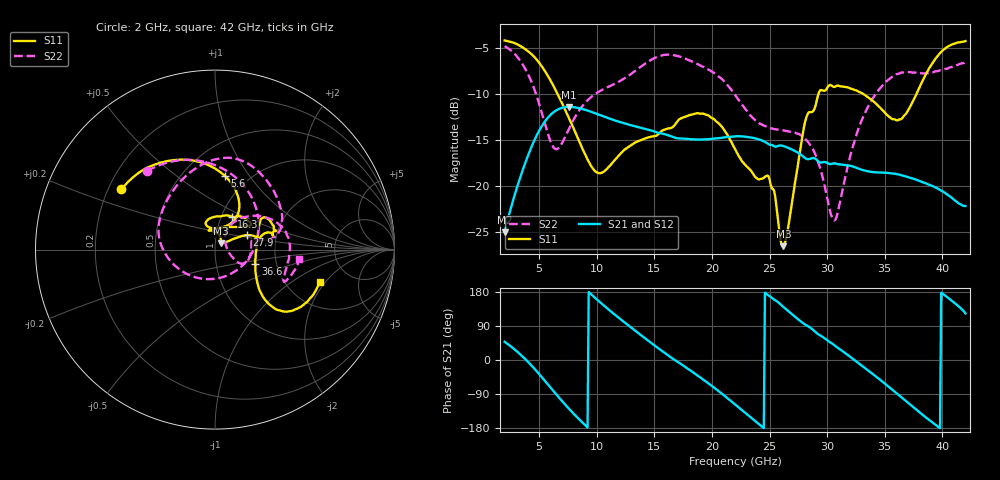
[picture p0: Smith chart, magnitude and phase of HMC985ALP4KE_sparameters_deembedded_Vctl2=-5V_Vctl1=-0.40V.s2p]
!s2p File: Measurements: S11, S21, S12, S22
# GHz S dB R 50.0
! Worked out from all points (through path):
!   401 points, 2 GHz to 42 GHz, reference 50 ohm
!   highest |S21| = -11.37 dB at 7.6 GHz (marker M1); lowest = -25.0 dB at 2 GHz (marker M2)
!   lowest |S11| = -26.5 dB at 26.2 GHz (marker M3), VSWR 1.10, Z = 53.2 + j3.72 ohm
!   |S11| at or under -10 dB: 6.609 GHz to 29.24 GHz (22.63 GHz wide, 126 % of centre); 33.17 GHz to 37.74 GHz (4.569 GHz wide, 12.9 % of centre)
!   |S22| runs from -23.7 to -4.8 dB; largest |S21 - S12| = 0.00026
!   S11 on the Smith chart (normalised r, x): 2 GHz: 0.25, +0.28; 5.6 GHz: 0.78, +0.77; 16.3 GHz: 1.12, +0.43; 27.9 GHz: 1.41, +0.24; 36.6 GHz: 1.55, -0.27; 42 GHz: 3.06, -1.79
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2  -4.15 147.2  -25.02 48.0  -25.02 48.1  -4.76 130.7
3.6  -4.93 120.5  -18.14 8.0  -18.14 8.0  -6.83 85.4
5.6  -7.68 82.1  -12.79 -58.7  -12.79 -58.7  -13.63 -4.5
6.5  -9.73 67.2  -11.73 -91.3  -11.74 -91.3  -15.96 -72.2
7.6  -12.62 57.1  -11.37 -129.1  -11.38 -129.1  -13.72 -138.4
8.7  -15.76 60.1  -11.58 -163.4  -11.59 -163.4  -11.36 -171.9
10.1  -18.54 86.0  -12.17 157.3  -12.18 157.3  -9.77 165.2
11.9  -16.68 109.8  -12.98 111.5  -12.98 111.6  -8.64 140.8
15.4  -14.28 76.8  -14.22 29.8  -14.22 29.8  -5.87 87.0
16.3  -13.71 62.9  -14.49 9.8  -14.49 9.9  -5.70 76.1
19.4  -12.19 34.8  -14.90 -55.0  -14.91 -55.0  -7.13 35.5
22  -15.94 52.3  -14.57 -117.1  -14.57 -117.1  -10.05 10.7
24.9  -18.91 102.1  -15.42 170.6  -15.42 170.6  -13.60 12.8
26.2  -26.52 47.6  -15.63 140.1  -15.63 140.1  -13.93 -1.9
27.9  -14.17 24.3  -16.75 97.4  -16.75 97.4  -14.60 -23.5
28.7  -11.92 12.2  -16.94 81.4  -16.95 81.4  -15.80 -28.5
30.7  -9.17 20.1  -17.52 37.2  -17.52 37.2  -23.67 23.7
32.9  -9.81 33.4  -18.17 -12.7  -18.17 -12.7  -13.14 51.3
35.4  -12.45 10.9  -18.57 -72.1  -18.58 -72.0  -8.34 21.5
36.6  -12.45 -19.8  -18.85 -102.5  -18.86 -102.4  -7.63 6.6
39.5  -5.99 -42.8  -20.19 -173.2  -20.19 -173.2  -7.49 -24.5
42  -4.22 -17.2  -22.15 122.8  -22.15 122.9  -6.49 -6.2
